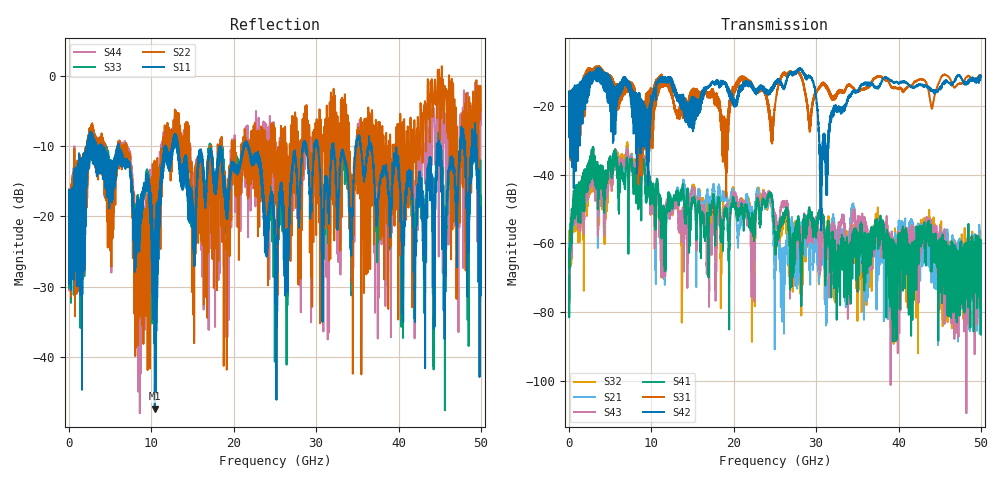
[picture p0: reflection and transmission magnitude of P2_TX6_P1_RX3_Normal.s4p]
!Keysight Technologies,N5225B,MY57041031,A.13.20.10
!Date: Friday, May 31, 2019 11:18:26
!Correction: S11(Full 4 Port(1,2,3,4))
!S12(Full 4 Port(1,2,3,4))
!S13(Full 4 Port(1,2,3,4))
!S14(Full 4 Port(1,2,3,4))
!S21(Full 4 Port(1,2,3,4))
!S22(Full 4 Port(1,2,3,4))
!S23(Full 4 Port(1,2,3,4))
!S24(Full 4 Port(1,2,3,4))
!S31(Full 4 Port(1,2,3,4))
!S32(Full 4 Port(1,2,3,4))
!S33(Full 4 Port(1,2,3,4))
!S34(Full 4 Port(1,2,3,4))
!S41(Full 4 Port(1,2,3,4))
!S42(Full 4 Port(1,2,3,4))
!S43(Full 4 Port(1,2,3,4))
!S44(Full 4 Port(1,2,3,4))
!S4P File: Measurements: <S11,S12,S13,S14>,
!<S21,S22,S23,S24>,
!<S31,S32,S33,S34>,
!<S41,S42,S43,S44>:
# Hz S  dB  R 50.0
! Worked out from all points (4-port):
!   5000 points, 10 MHz to 50 GHz, reference 50 ohm
!   strongest paths, dB at 10 MHz, 12.51 GHz, 25.01 GHz, 37.51 GHz, 50 GHz:
!     S42: -19.6, -14.3, -13.5, -14.6, -11.2
!     S31: -19.3, -16.8, -20.0, -11.6, -11.4
!     S41: -69.6, -48.3, -57.0, -58.0, -60.2
!     S43: -66.8, -50.1, -51.1, -54.9, -62.3
!     S21: -60.0, -48.9, -69.9, -63.0, -61.9
!     S32: -56.4, -50.7, -56.8, -52.6, -66.8
!   lowest |S11| = -47.4 dB at 10.41 GHz (marker M1), VSWR 1.01, Z = 50.1 - j0.424 ohm
!   |S11| at or under -10 dB: 13.21 GHz to 21.18 GHz (7.966 GHz wide, 46.3 % of centre); 21.74 GHz to 28.38 GHz (6.638 GHz wide, 26.5 % of centre); 36.67 GHz to 44.63 GHz (7.961 GHz wide, 19.6 % of centre)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
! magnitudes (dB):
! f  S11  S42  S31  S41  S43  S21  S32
! 10 MHz  -19.3  -19.6  -19.3  -69.6  -66.8  -60.0  -56.4
! 2.74 GHz  -10.7  -13.6  -12.1  -33.3  -34.0  -33.8  -34.5
! 10.41 GHz  -47.4  -15.7  -14.8  -52.3  -61.6  -52.8  -61.7
! 12.81 GHz  -8.3  -15.4  -19.8  -47.4  -49.1  -46.3  -48.3
! 28.07 GHz  -15.6  -9.1  -10.9  -61.7  -62.2  -57.2  -68.6
! 30.63 GHz  -19.1  -40.3  -13.7  -52.4  -58.4  -66.4  -58.1
! 50 GHz  -23.2  -11.2  -11.4  -60.2  -62.3  -61.9  -66.8
